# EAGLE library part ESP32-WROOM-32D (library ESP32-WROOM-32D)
Bluetooth, WiFi 802.11b/g/n, Bluetooth v4.2 + EDR, Class 1, 2 and 3 Transceiver Module 2.4GHz ~ 2.5GHz Integrated, Trace Surface Mount
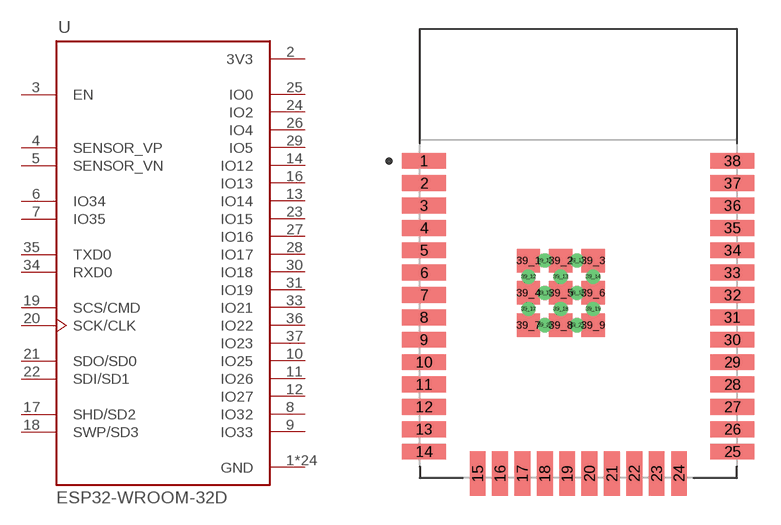
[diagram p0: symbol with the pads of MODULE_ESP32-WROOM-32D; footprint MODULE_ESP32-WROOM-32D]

Designator prefix U

## ESP32-WROOM-32D (AVAILABILITY: Unavailable; DESCRIPTION: Bluetooth, WiFi 802.11b/g/n, Bluetooth v4.2 +EDR, Class 1, 2 and 3 Transceiver Module 2.4GHz ~ 2.5GHz Integrated, Trace Surface Mount; MF: Espressif Systems; MP: ESP32-WROOM-32D; PACKAGE: Module Espressif Systems; PRICE: None)  [MODULE_ESP32-WROOM-32D]
1  GND  pwr
2  3V3  pwr
3  EN  in
4  SENSOR_VP  in
5  SENSOR_VN  in
6  IO34  in
7  IO35  in
8  IO32
9  IO33
10  IO25
11  IO26
12  IO27
13  IO14
14  IO12
15  GND  pwr
16  IO13
17  SHD/SD2
18  SWP/SD3
19  SCS/CMD
20  SCK/CLK
21  SDO/SD0
22  SDI/SD1
23  IO15
24  IO2
25  IO0
26  IO4
27  IO16
28  IO17
29  IO5
30  IO18
31  IO19
33  IO21
34  RXD0
35  TXD0
36  IO22
37  IO23
38  GND  pwr
39_1  GND  pwr
39_2  GND  pwr
39_3  GND  pwr
39_4  GND  pwr
39_5  GND  pwr
39_6  GND  pwr
39_7  GND  pwr
39_8  GND  pwr
39_9  GND  pwr
39_10  GND  pwr
39_11  GND  pwr
39_12  GND  pwr
39_13  GND  pwr
39_14  GND  pwr
39_15  GND  pwr
39_16  GND  pwr
39_17  GND  pwr
39_18  GND  pwr
39_19  GND  pwr
39_20  GND  pwr
39_21  GND  pwr

## Footprint MODULE_ESP32-WROOM-32D (pad centres in mm)
smd 2.5 x 0.9: 1 -8.75,5.26; 2 -8.75,3.99; 3 -8.75,2.72; 4 -8.75,1.45; 5 -8.75,0.18; 6 -8.75,-1.09; 7 -8.75,-2.36; 8 -8.75,-3.63; 9 -8.75,-4.9; 10 -8.75,-6.17; 11 -8.75,-7.44; 12 -8.75,-8.71; 13 -8.75,-9.98; 14 -8.75,-11.25; 25 8.75,-11.25; 26 8.75,-9.98; 27 8.75,-8.71; 28 8.75,-7.44; 29 8.75,-6.17; 30 8.75,-4.9; 31 8.75,-3.63; 32 8.75,-2.36; 33 8.75,-1.09; 34 8.75,0.18; 35 8.75,1.45; 36 8.75,2.72; 37 8.75,3.99; 38 8.75,5.26
smd 0.9 x 2.5: 15 -5.715,-12.5; 16 -4.445,-12.5; 17 -3.175,-12.5; 18 -1.905,-12.5; 19 -0.635,-12.5; 20 0.635,-12.5; 21 1.905,-12.5; 22 3.175,-12.5; 23 4.445,-12.5; 24 5.715,-12.5
smd 1.33 x 1.33: 39_1 -2.835,-0.405; 39_2 -1,-0.405; 39_3 0.835,-0.405; 39_4 -2.835,-2.24; 39_5 -1,-2.24; 39_6 0.835,-2.24; 39_7 -2.835,-4.075; 39_8 -1,-4.075; 39_9 0.835,-4.075
drill 0.3 pad 0.4: 39_10 -1.917,-0.405; 39_11 -0.083,-0.405; 39_12 -2.835,-1.323; 39_13 -1,-1.323; 39_14 0.835,-1.323; 39_15 -1.917,-2.24; 39_16 -0.083,-2.24; 39_17 -2.835,-3.158; 39_18 -1,-3.158; 39_19 0.835,-3.158; 39_20 -1.917,-4.075; 39_21 -0.083,-4.075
